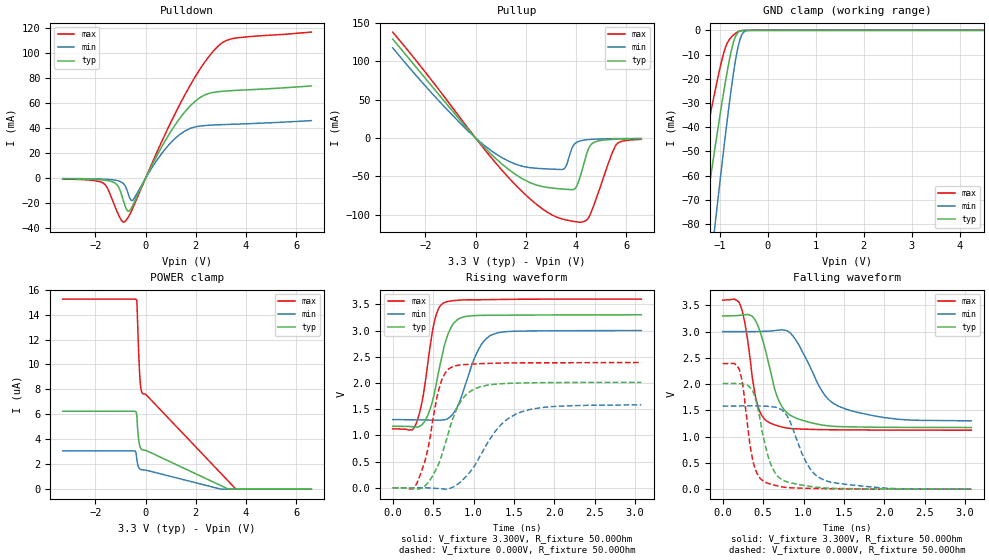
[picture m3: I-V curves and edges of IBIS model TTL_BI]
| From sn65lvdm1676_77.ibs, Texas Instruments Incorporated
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|   Receiver Output/Driver Input Model
[Model]   TTL_BI
Model_type   3-state
| Signals   A1A,A2A,A3A,A4A,B1A,B2A,B3A,B4A,C1A,C2A,C3A,C4A,D1A,D2A,D3A,D4A
Vmeas = 1.5V   |Reference voltage for timing measurements
Cref  = 10pF   |Timing specification test load capacitance value
Vref  = 0V   |Timing specification test load voltage; GND
Rref  = 100
| variable   typ   min   max
|ccomp in RCV mode
C_comp   3.679pF   3.756pF   3.537pF
|ccomp in DRV mode
|C_comp   3.592pF   4.157pF   2.599pF
| Junction Temperature (Ambient temp is 25C typ, 85C min, 0C max)
[Temperature Range]   40.0   100   -40
[Voltage range]   3.3V   3.0V   3.6V
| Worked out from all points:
|   slope of the pulldown table from 0 to 0.495 V, typ, clamps not added: 25.2 ohm
|   slope of the pullup table from 0 to 0.495 V, typ, clamps not added: 29.1 ohm
|   GND clamp passes 1 mA (typ) near -0.63 V on its own axis
|   falling waveform, V_fixture 3.300V, R_fixture 50.00Ohm: 20-80 % time 236ps typ, 394ps min, 148ps max; typ from 3.3 V to 1.17 V
|   rising waveform, V_fixture 3.300V, R_fixture 50.00Ohm: 20-80 % time 189ps typ, 243ps min, 146ps max; typ from 1.17 V to 3.3 V
|   rising waveform, V_fixture 0.000V, R_fixture 50.00Ohm: 20-80 % time 274ps typ, 421ps min, 187ps max; typ from 0 V to 2.01 V
|   falling waveform, V_fixture 0.000V, R_fixture 50.00Ohm: 20-80 % time 192ps typ, 281ps min, 130ps max; typ from 2.01 V to 0 V
[Pulldown]
|   Voltage   I(typ)   I(min)   I(max)
-3.3V     -440uA     -266.7uA   -669.7uA
-1.662V   -1.517mA   -793.7uA   -4.286mA
-1.141V   -5.204mA   -1.849mA   -26.4mA
-843.6mV  -20.58mA   -5.295mA   -35.08mA
-694.7mV  -26.42mA   -12.36mA   -31.35mA
-521.1mV  -22.08mA   -17.76mA   -24.52mA
446.6mV   17.84mA    14.27mA    20.57mA
1.191V    43.03mA    32.06mA    52.29mA
2.01V     62.15mA    41.19mA    82.29mA
2.804V    69mA       42.67mA    104mA
3.523V    70.21mA    43.2mA     112mA
6.6V      73.83mA    46.08mA    117mA
[GND Clamp]
|   Voltage   I(typ)   I(min)   I(max)
-3.3V     -360.9mA   -499.6mA   -260.5mA
-1.662V   -125.1mA   -183.5mA   -82.71mA
-1.613V   -118.2mA   -174.2mA   -77.47mA
-1.34V    -80.49mA   -123.6mA   -49mA
-1.117V   -50.47mA   -83.28mA   -26.59mA
-1.092V   -47.21mA   -78.88mA   -24.2mA
-918mV    -25.26mA   -48.85mA   -9.215mA
-794mV    -11.47mA   -28.86mA   -3.586mA
-694.7mV  -3.562mA   -14.85mA   -1.543mA
-595.5mV  -483.9uA   -4.76mA    -373.8uA
-397mV    -4.467uA   -35.79uA   -4.25uA
6.6V      0A         0A         0A
[Pullup]
|   Voltage   I(typ)   I(min)   I(max)
-3.3V     129.1mA    117.6mA    138.1mA
-1.117V   43mA       36.46mA    48.23mA
521.1mV   -17.88mA   -14.01mA   -21.47mA
1.935V    -54.33mA   -37.3mA    -72.33mA
3.226V    -65.82mA   -40.82mA   -103mA
3.573V    -66.78mA   -38.28mA   -106.6mA
3.821V    -67.27mA   -14.66mA   -108.2mA
3.97V     -65.56mA   -6.918mA   -109mA
4.441V    -18.95mA   -2.18mA    -106.3mA
4.739V    -5.305mA   -1.495mA   -84.81mA
5.608V    -1.561mA   -772.1uA   -8.37mA
6.6V      -859.5uA   -494.9uA   -1.675mA
[POWER Clamp]
|   Voltage   I(typ)   I(min)   I(max)
-3.3V     6.251uA    3.069uA    15.25uA
-471.4mV  6.25uA     3.068uA    15.25uA
-372.2mV  6.184uA    2.845uA    15.21uA
-347.4mV  5.891uA    2.38uA     15.13uA
-297.7mV  4.38uA     1.874uA    12.2uA
-248.1mV  3.621uA    1.666uA    9.687uA
-223.3mV  3.424uA    1.616uA    8.819uA
-198.5mV  3.301uA    1.584uA    8.25uA
-148.9mV  3.182uA    1.553uA    7.76uA
3.3V      0A         0A         630.9nA
3.598V    0A         0A         0A
6.6V      0A         0A         0A
[Ramp]
R_load = 50.00Ohm
|   typ   min   max
dV/dt_r   1.207V/273.965ps 949.546mV/420.301ps   1.434V/186.039ps
dV/dt_f   1.276V/235.644ps   1.019V/394.089ps   1.486V/147.287ps
[Falling Waveform]
V_fixture = 3.300V
V_fixture_min = 3.000V
V_fixture_max = 3.600V
R_fixture = 50.00Ohm
|   Time   V(typ)   V(min)   V(max)
0s        3.3V       3V         3.6V
219ps     3.31V      3V         3.499V
287ps     3.323V     2.999V     3.051V
420ps     3.165V     3V         1.666V
577ps     2.34V      3.01V      1.267V
677ps     1.75V      3.025V     1.208V
807ps     1.441V     3.007V     1.162V
1.239ns   1.22V      1.845V     1.133V
1.432ns   1.192V     1.58V      1.129V
3.077ns   1.174V     1.301V     1.123V
[Rising Waveform]
V_fixture = 3.300V
V_fixture_min = 3.000V
V_fixture_max = 3.600V
R_fixture = 50.00Ohm
|   Time   V(typ)   V(min)   V(max)
0s        1.174V     1.301V     1.123V
290ps     1.159V     1.297V     1.223V
372ps     1.218V     1.295V     1.714V
514ps     1.792V     1.292V     3.157V
630ps     2.648V     1.296V     3.528V
713ps     3.03V      1.357V     3.561V
810ps     3.215V     1.579V     3.578V
1.043ns   3.286V     2.579V     3.586V
1.216ns   3.291V     2.91V      3.59V
3.077ns   3.3V       3V         3.6V
[Rising Waveform]
V_fixture = 0.000V
V_fixture_min = 0.000V
V_fixture_max = 0.000V
R_fixture = 50.00Ohm
|   Time   V(typ)   V(min)   V(max)
0s        511.1pV    3.401nV    257.3pV
299ps     -23.3mV    444.8uV    89.64mV
423ps     72.13mV    -1.241mV   660.2mV
584ps     518.5mV    -16.44mV   1.947V
739ps     1.295V     7.795mV    2.31V
851ps     1.666V     128.5mV    2.346V
981ps     1.86V      349.2mV    2.359V
1.289ns   1.979V     1.115V     2.378V
1.556ns   1.999V     1.426V     2.383V
3.077ns   2.011V     1.583V     2.39V
[Falling Waveform]
V_fixture = 0.000V
V_fixture_min = 0.000V
V_fixture_max = 0.000V
R_fixture = 50.00Ohm
|   Time   V(typ)   V(min)   V(max)
0s        2.011V     1.583V     2.39V
202ps     2.009V     1.584V     2.29V
248ps     2V         1.584V     1.98V
375ps     1.853V     1.586V     535.8mV
525ps     846.6mV    1.58V      134.2mV
697ps     221.8mV    1.537V     55.38mV
821ps     127.4mV    1.328V     27.85mV
1.046ns   61.71mV    477mV      16.73mV
1.216ns   28.33mV    199.7mV    11.14mV
3.077ns   511.1pV    3.401nV    257.3pV
